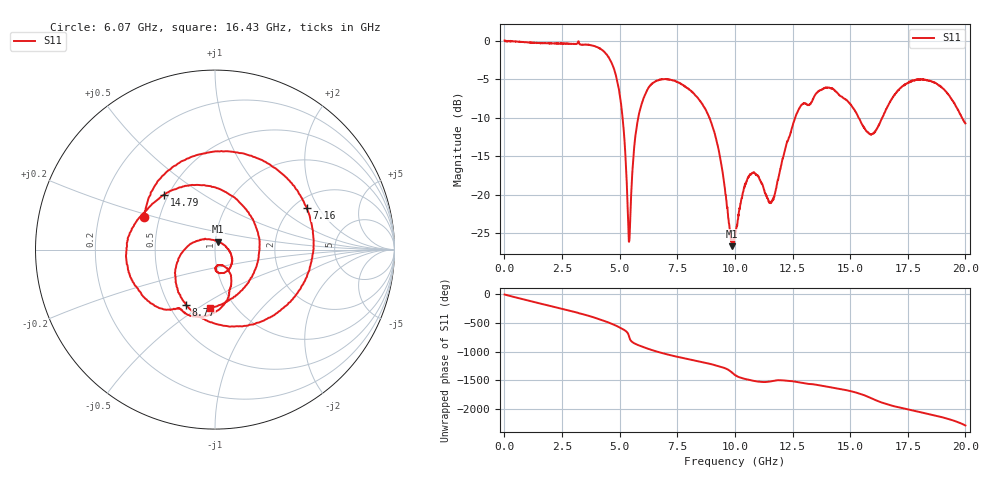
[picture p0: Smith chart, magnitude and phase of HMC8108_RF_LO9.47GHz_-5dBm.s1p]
! Analog Devices, Inc.
! 1 Analog Way
! Wilmington, MA 01887
! http://www.analog.com
! Date:  2021-09-07 NN
! Board Name:  EV1HMC8108LC5 Revision A with HMC8108LC5 installed
! File Description:  S-Parameters for evaluation board without connectors or board loss de-embedded
! File Generation:  Calibrated Network Analyzer
! Chip Part Number:  HMC8108
! Chip Description:  X-Band, GaAs, MMIC, Low Noise Converter
! Chip Frequency:  9 to 10 GHz
! Chip Package:  LCC, 5 x 5 x 1.12 mm
! Chip State:
!  Temperature:  25C
!  LO Frequency:  9.47GHz
!  LO Power:  -5dBm
! Note:
!  Analog Devices supplies this data as a sample of measured data at the evaluation board
!  ports for this product.  Your particular data for this product may vary.
!  Analog Devices reserves the right to change this data at anytime.
!  All lines below in this file are as is from the Network Analyzer.
!Keysight Technologies,N5245A,MY49151104,A.10.65.16
!Date: Thursday, August 19, 2021 13:44:22
!Correction: S11(Full 2 Port(1,2))
!S1P File: Measurement: S11:
# Hz S  dB  R 50
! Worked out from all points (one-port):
!   2000 points, 10 MHz to 20 GHz, reference 50 ohm
!   lowest |S11| = -26.7 dB at 9.89 GHz (marker M1), VSWR 1.10, Z = 51.4 + j4.49 ohm
!   |S11| at or under -10 dB: 5.128 GHz to 5.807 GHz (678.7 MHz wide, 12.4 % of centre); 8.895 GHz to 12.61 GHz (3.718 GHz wide, 34.6 % of centre); 15.37 GHz to 16.39 GHz (1.018 GHz wide, 6.41 % of centre)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
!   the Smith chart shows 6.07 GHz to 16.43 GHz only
!   S11 on the Smith chart (normalised r, x): 6.07 GHz: 0.41, +0.19; 7.16 GHz: 2.33, +1.58; 8.77 GHz: 0.61, -0.43; 14.79 GHz: 0.47, +0.35; 16.43 GHz: 0.77, -0.56
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1e7  0.06 -1.5
5.6e8  -0.10 -59.0
9.9e8  -0.17 -102.7
1.75e9  -0.31 -177.5
2.51e9  -0.35 108.7
2.97e9  -0.40 62.2
3.46e9  -0.49 9.6
4.17e9  -1.04 -78.1
4.64e9  -2.79 -149.0
5.01e9  -7.07 143.1
5.42e9  -25.96 -29.8
6.07e9  -7.24 155.1
6.58e9  -5.24 87.4
7.16e9  -5.03 24.5
7.51e9  -5.36 -8.8
8.77e9  -9.14 -117.6
9.89e9  -26.70 70.6
1.001e10  -25.43 33.3
1.251e10  -10.97 -75.5
1.398e10  -6.07 -167.7
1.479e10  -7.60 132.9
1.501e10  -8.21 113.3
1.579e10  -11.91 12.4
1.643e10  -9.74 -94.5
1.751e10  -5.46 152.8
1.825e10  -5.04 87.8
1.898e10  -6.06 18.3
2e10  -10.73 -126.2
